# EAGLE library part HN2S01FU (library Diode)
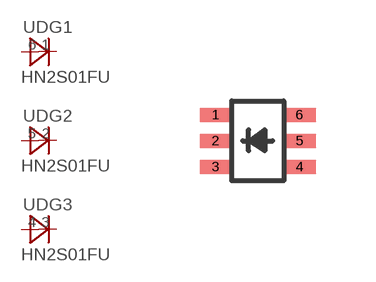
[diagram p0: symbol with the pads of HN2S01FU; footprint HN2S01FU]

Designator prefix UD; gates G1=DIODE G2=DIODE G3=DIODE

## HN2S01FU  [HN2S01FU]
1  G1:C  pas
2  G2:C  pas
3  G3:C  pas
4  G3:A  pas
5  G2:A  pas
6  G1:A  pas

## Footprint HN2S01FU (pad centres in mm)
smd 0.8 x 0.35: 1 -1.05,0.65; 2 -1.05,0; 3 -1.05,-0.65; 4 1.05,-0.65; 5 1.05,0; 6 1.05,0.65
